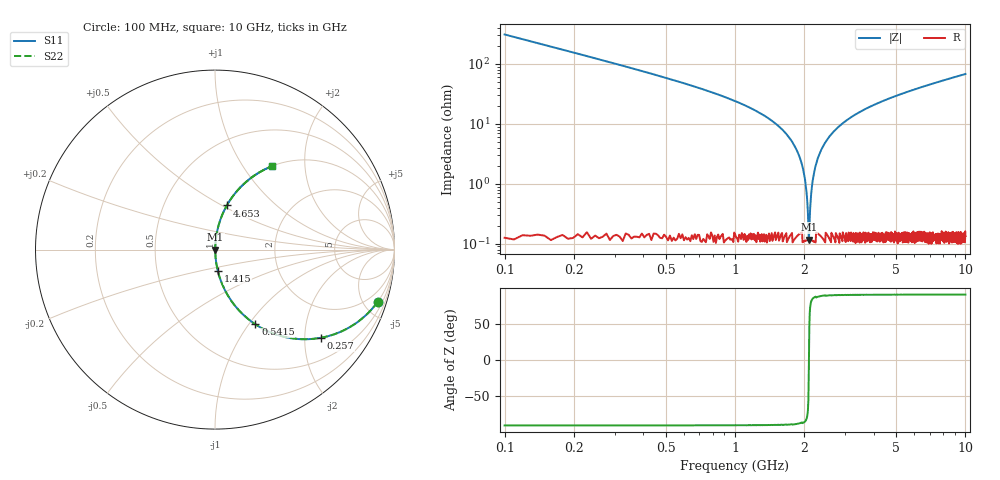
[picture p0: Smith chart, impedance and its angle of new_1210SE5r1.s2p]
!	AVX	Thin	Film	Operation	Date:	April 2007
!	Description:	Accu-P®	"Series,"	Thin	"Film,"	"SMD,"	RF	Capacitor
!	Part	Number:	12101J5R1ABT
!	100	MHz	-	5.05	GHz
!	Serial	Measurements
#	MHZ	S	MA	R	50
!	S11	S21	S12	S22
!	dB	Phase	dB	Phase	dB	Phase	dB	Phase
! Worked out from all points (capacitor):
!   1010 points, 100 MHz to 10 GHz, reference 50 ohm
!   read as one part in series: C = 5.1 pF near 149.1 MHz
!   lowest |Z| = 118 mohm at 2.092 GHz (marker M1)
!   series resonance near 2.094 GHz, so ESL is about 1.1 nH
!   S11 on the Smith chart (normalised r, x): 100 MHz: 1.00, -6.23; 257 MHz: 1.00, -2.39; 541.5 MHz: 1.00, -1.08; 1.415 GHz: 1.00, -0.24; 4.653 GHz: 1.00, +0.53; 10 GHz: 1.00, +1.36
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100  0.952 -17.8  0.306 72.2  0.306 72.2  0.952 -17.8
256.987  0.767 -39.9  0.641 50.1  0.641 50.1  0.767 -39.9
541.526  0.473 -61.6  0.88 28.2  0.88 28.2  0.473 -61.6
875.124  0.282 -73.4  0.958 16.4  0.958 16.4  0.282 -73.4
1414.767  0.119 -82.6  0.992 6.8  0.992 6.8  0.119 -82.6
1758.176  0.052 -85.6  0.997 3.0  0.997 3.0  0.052 -85.6
1964.222  0.019 -85.0  0.999 1.1  0.999 1.1  0.019 -85.0
2013.28  0.012 -83.0  0.999 0.7  0.999 0.7  0.012 -83.0
2062.339  0.00466 -73.6  0.999 0.3  0.999 0.3  0.00466 -73.6
2091.774  0.00132 -11.0  0.999 0.0  0.999 0.0  0.00132 -11.0
2131.021  0.00544 75.9  0.999 -0.3  0.999 -0.3  0.00544 75.9
2170.268  0.011 82.5  0.999 -0.6  0.999 -0.6  0.011 82.5
2219.326  0.017 84.7  0.999 -1.0  0.999 -1.0  0.017 84.7
2297.82  0.028 85.7  0.998 -1.6  0.998 -1.6  0.028 85.7
2415.56  0.043 85.8  0.998 -2.4  0.998 -2.4  0.043 85.8
2768.781  0.084 84.3  0.995 -4.8  0.995 -4.8  0.084 84.3
3406.541  0.149 80.9  0.988 -8.6  0.988 -8.6  0.149 80.9
4652.626  0.255 74.9  0.966 -14.8  0.966 -14.8  0.255 74.9
5054.906  0.285 73.2  0.957 -16.6  0.957 -16.6  0.285 73.2
6703.271  0.395 66.6  0.917 -23.3  0.917 -23.3  0.395 66.6
8351.635  0.486 60.8  0.873 -29.1  0.873 -29.1  0.486 60.8
10000  0.562 55.7  0.826 -34.2  0.826 -34.2  0.562 55.7
